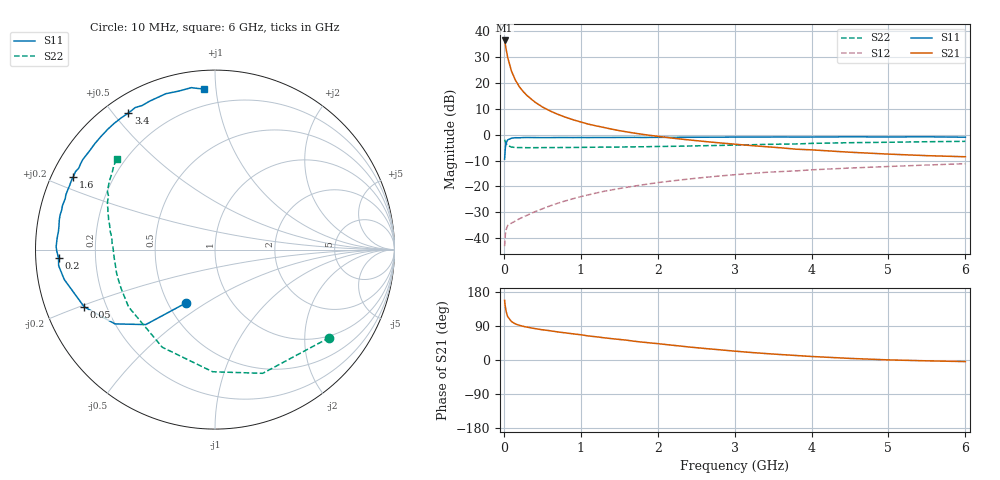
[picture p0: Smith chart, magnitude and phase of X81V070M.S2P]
! SIEMENS Small Signal Semiconductors
! BFP136W
! Si NPN RF Bipolar Junction Transistor in SOT343
! VCE = 1 V  IC = 70 mA
! Common Emitter S-Parameters:  September  1994
# GHz  S  MA  R  50
!  f  S11  S21  S12  S22
! GHz  MAG  ANG  MAG  ANG  MAG  ANG  MAG  ANG
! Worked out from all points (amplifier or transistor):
!   40 points, 10 MHz to 6 GHz, reference 50 ohm
!   highest |S21| = 36.5 dB at 10 MHz (marker M1)
!   |S21| within 3 dB of that: start of sweep to 27.87 MHz
!   unconditionally stable (mu >= 1): 473.4 MHz to 3.257 GHz; 3.733 GHz to 3.904 GHz; 5.865 GHz to end of sweep
!   at 200 MHz: K = 0.67, MSG = 25.6 dB, |S12| = -32.5 dB
!   at 1.5 GHz: K = 1.12, MAG = 9.1 dB, |S12| = -20.8 dB
!   at 6 GHz: K = 1.02, MAG = 0.6 dB, |S12| = -11.2 dB
!   S11 on the Smith chart (normalised r, x): 10 MHz: 0.62, -0.41; 50 MHz: 0.12, -0.21; 200 MHz: 0.07, -0.03; 1.6 GHz: 0.06, +0.24; 3.4 GHz: 0.07, +0.55; 6 GHz: 0.10, +0.93
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0.01  0.3379 -118.5  66.55 157.3  0.007 66.0  0.8041 -37.6
0.02  0.5683 -132.7  55.23 139.7  0.012 52.5  0.7389 -68.9
0.03  0.6943 -143.4  45.12 127.8  0.0146 44.1  0.6807 -91.1
0.05  0.7958 -156.4  31.21 114.4  0.0176 34.4  0.6183 -118.4
0.1  0.8564 -168.8  16.86 101.2  0.0196 31.2  0.5778 -146.5
0.15  0.8756 -174.1  11.4 95.2  0.0214 34.5  0.566 -157.7
0.2  0.8731 -176.9  8.542 91.6  0.0236 37.8  0.564 -163.5
0.25  0.8814 -179.4  6.884 88.9  0.0256 41.0  0.5636 -167.2
0.3  0.8853 179.0  5.752 86.8  0.0276 44.5  0.5618 -169.8
0.4  0.8817 175.8  4.326 83.0  0.0323 49.3  0.5622 -173.1
0.5  0.8781 173.3  3.452 79.8  0.0369 52.7  0.5635 -175.5
0.6  0.879 171.5  2.885 77.2  0.0421 55.1  0.5643 -177.1
0.7  0.8835 169.0  2.488 74.1  0.0473 57.2  0.5653 -178.4
0.9  0.8822 165.5  1.949 69.0  0.0579 58.8  0.5675 179.2
1.1  0.8816 161.2  1.602 63.4  0.0688 59.6  0.5715 177.5
1.6  0.8878 152.7  1.133 52.2  0.0963 58.5  0.5807 173.4
2.2  0.8893 142.4  0.856 38.8  0.1286 54.0  0.5972 168.4
3.2  0.9009 125.4  0.62 20.1  0.1773 44.3  0.6388 159.1
3.4  0.9011 122.4  0.588 17.1  0.1872 42.1  0.6508 157.2
4.5  0.9108 107.5  0.459 4.2  0.227 31.7  0.7015 147.1
5.5  0.912 98.3  0.394 -2.2  0.2596 23.7  0.7327 140.3
6  0.8958 94.0  0.375 -4.2  0.2755 19.3  0.7448 137.3
